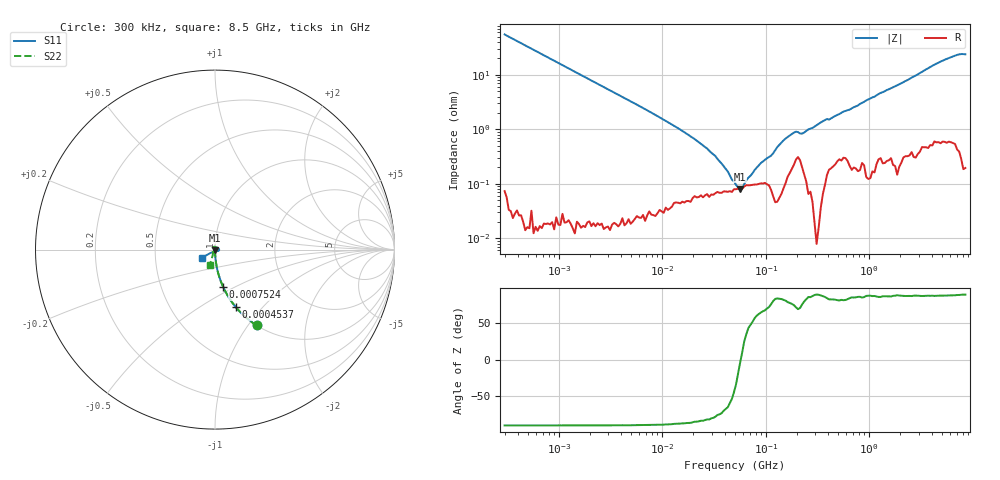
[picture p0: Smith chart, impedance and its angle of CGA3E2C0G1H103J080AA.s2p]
! S-parameter Generated by TDK Corporation
! Copyright(C) 2015 TDK Corporation.
! All Rights Reserved.
! TDK P/N: CGA3E2C0G1H103J080AA (Multilayer Ceramic Chip Capacitors)
! Property: C=10nF
! Size(LxWxT): 1.6x0.8x0.8mm, 0.063x0.031x0.031inches
! Model Type: s2p (Touchstone File Format Version 1.0)
! Frequency: DC=Yes Start=0.3MHz Stop=8500MHz 225points Log-sweep
! Note:
! Model Generated on Jun. 23, 2015
! Hash(MD5):
! Port Assignments:
!  1 ---| |--- 2
! Applicable Conditions:
!  Temperature = 25 degC
!  DC Bias Voltage = 0 V
!  Small Signal Operation
! Terms and conditions regarding TDK Simulation Models
! (1)This simulation model is being provided solely for informational purposes. Please refer to the specifications of the products in terms of detailed characteristics of such products.
! (2)In no event shall TDK Corporation of any of its subsidiaries be liable for any loss or damage arising, directly or indirectly,
!  From any information contained in this simulation model, including, but not limited to loss or damages arising from any inaccuracies, omissions or errors in connection with such information.
! (3)Any and all copyrights on this simulation model are owned by TDK Corporation.
!  Duplication or redistribution of this simulation model without prior written permission from TDK Corporation is prohibited.
! (4)This simulation model is subject to any modification or change without any prior notice.
! (5)Neither TDK Corporation nor any of its subsidiaries shall make any warranty, express or implied,
!  Including but not limited to the correctness, implied warranties of merchantability and fitness for a particular purpose with respect to this simulation models.
! (6)The use of this simulation model shall be deemed to have consented to the terms and conditions hereof.
# MHz S MA R 50
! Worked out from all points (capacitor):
!   224 points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, 300 kHz to 8.5 GHz, reference 50 ohm
!   read as one part in series: C = 9.66 nF near 314.1 kHz
!   lowest |Z| = 80.9 mohm at 56.65 MHz (marker M1)
!   series resonance near 57.33 MHz, so ESL is about 800 pH
!   S11 on the Smith chart (normalised r, x): 300 kHz: 1.00, -1.10; 453.7 kHz: 1.00, -0.73; 752.4 kHz: 1.00, -0.44; 8.5 GHz: 0.86, -0.08
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0.3  0.4821 -61.1  0.8761 28.7  0.8761 28.9  0.4821 -61.2
0.4537435  0.341 -70.1  0.9395 19.9  0.9397 20.0  0.3406 -70.1
0.7523683  0.2132 -77.7  0.9768 12.3  0.9769 12.4  0.213 -77.6
1.72111  0.09488 -84.5  0.9954 5.4  0.9953 5.5  0.09485 -84.5
9.430415  0.01694 -88.0  0.9995 0.9  0.9996 1.0  0.01701 -88.0
51.67171  0.002204 -76.7  0.9985 -0.1  0.9993 -0.0  0.002576 -79.3
56.64789  0.001905 -74.8  0.9985 -0.1  0.9993 -0.1  0.002282 -76.5
112.8926  0.0008278 -50.9  0.9987 -0.4  0.9994 -0.4  0.0009504 -41.3
129.5872  0.0001695 54.6  0.9992 -0.5  0.9997 -0.5  0.0007231 21.1
178.7805  0.002737 61.9  0.9977 -0.8  0.9984 -0.8  0.002437 19.3
283.1228  0.003259 147.0  0.9971 -1.2  0.9978 -1.2  0.001078 -117.2
564.2308  0.002432 43.0  0.996 -2.3  0.997 -2.3  0.003937 29.9
778.4218  0.0002921 -71.3  0.9965 -3.1  0.9974 -3.1  0.0006687 -15.7
893.5346  0.002741 45.9  0.997 -3.7  0.9969 -3.6  0.001891 -60.8
1073.923  0.0005805 132.5  0.995 -4.3  0.9969 -4.4  0.001364 132.4
1290.729  0.003115 44.2  0.9956 -5.3  0.9957 -5.2  0.001473 25.9
1551.304  0.0004777 -31.4  0.9948 -6.3  0.9955 -6.2  0.00112 8.3
2044.041  0.004149 -101.3  0.9948 -8.2  0.9956 -8.3  0.001968 -93.6
3237.012  0.00155 145.9  0.9933 -13.1  0.9937 -13.0  0.00827 0.2
4465.833  0.01572 48.3  0.9913 -17.9  0.9919 -17.8  0.0144 67.3
7072.242  0.01008 -72.2  0.9891 -28.3  0.9894 -28.2  0.01425 -152.0
8500  0.08813 -147.8  0.9843 -33.9  0.9859 -34.0  0.09296 -108.7
